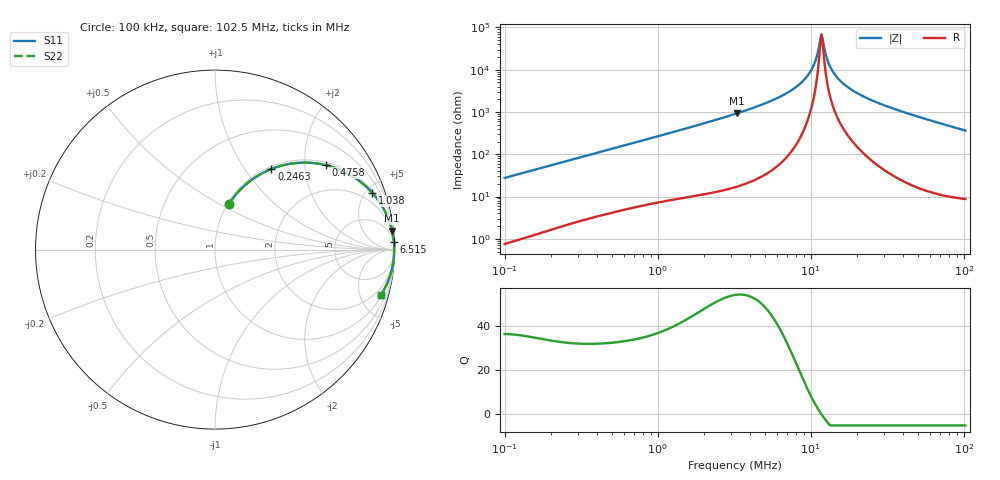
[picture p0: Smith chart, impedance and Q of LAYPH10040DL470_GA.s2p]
! LAYPH10040DL470_GA  S-PARAMETER MODEL  ( General Type )
! Model Generated by TAIYO YUDEN Corporation (http://www.ty-top.com)
! Version 1.0
! TAIYO YUDEN Control No. 180920NI43SB-FBB
! Copyright(c) 2018 TAIYO YUDEN CO.,LTD. All Rights Reserved.
! Product Description (link to TY-COMPAS)
! https://ds.yuden.co.jp/TYCOMPAS/or/detail?pn=LAYPH10040DL470MGA&u=M
! Products Name : Inductors
! Characteristics :
!  Inductance : 47 uH , SRF(min) : -Hz , DC Resistance(max) : 0.162 Ohm
!  Rated Current : Saturation :1.7 A , Temp Rise : 0.76 A (25 degC)
!  Case Size : 10.1 x 10.0 / 0.398 x 0.394 [mm/inch] , Thickness : 4 / 0.157 [mm/inch]
!  (Conditions: Temperature = 25 degC , DC Bias Current/Voltage = 0A / 0V)
! External Node Assignments :
!  1  o---GGG---o  2
! GND o---------o GND
! Frequency Range : 0.1MHz  -  102.47202MHz  [ 402 STEP ]
# MHz S RI R 50
! Freq[MHz].  S11 Real  S11 Imag  S21 Real  S21 Imag  S12 Real  S12 Imag  S22 Real  S22 Imag
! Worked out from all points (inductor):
!   401 points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, 100 kHz to 102.5 MHz, reference 50 ohm
!   read as one part in series: L = 43.7 uH near 103.5 kHz
!   highest Q = 54.3 at 3.314 MHz (marker M1), where L = 44.9 uH
!   self-resonance near 11.74 MHz
!   S11 on the Smith chart (normalised r, x): 100 kHz: 1.02, +0.55; 246.3 kHz: 1.04, +1.34; 475.8 kHz: 1.08, +2.55; 1.038 MHz: 1.15, +5.50; 6.515 MHz: 2, +49; 102.5 MHz: 1.17, -7.26
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0.1  0.0767 0.2527  0.9233 -0.2527  0.9233 -0.2527  0.0767 0.2527
0.246251  0.3147 0.4493  0.6853 -0.4493  0.6853 -0.4493  0.3147 0.4493
0.319357  0.4293 0.4796  0.5707 -0.4796  0.5707 -0.4796  0.4293 0.4796
0.475758  0.6159 0.4712  0.3841 -0.4712  0.3841 -0.4712  0.6159 0.4712
1.019889  0.8733 0.3194  0.1267 -0.3194  0.1267 -0.3194  0.8733 0.3194
1.037718  0.8769 0.3154  0.1231 -0.3154  0.1231 -0.3154  0.8769 0.3154
3.257086  0.9863 0.1074  0.0137 -0.1074  0.0137 -0.1074  0.9863 0.1074
3.314024  0.9868 0.1053  0.0132 -0.1053  0.0132 -0.1053  0.9868 0.1053
6.514629  0.9972 0.0408  0.00279 -0.0408  0.00279 -0.0408  0.9972 0.0408
8.596346  0.9984 0.0208  0.00156 -0.0208  0.00156 -0.0208  0.9984 0.0208
9.538344  0.9986 0.0137  0.00139 -0.0137  0.00139 -0.0137  0.9986 0.0137
10.22302  0.9986 0.00915  0.00136 -0.00915  0.00136 -0.00915  0.9986 0.00915
10.76858  0.9986 0.00575  0.00137 -0.00575  0.00137 -0.00575  0.9986 0.00575
11.54156  0.9986 0.00126  0.00143 -0.00126  0.00143 -0.00126  0.9986 0.00126
11.74333  0.9985 0.000148  0.00146 -0.000148  0.00146 -0.000148  0.9985 0.000148
12.1575  0.9985 -0.00208  0.00151 0.00208  0.00151 0.00208  0.9985 -0.00208
12.8063  0.9984 -0.00541  0.00161 0.00541  0.00161 0.00541  0.9984 -0.00541
13.48973  0.9983 -0.00875  0.00173 0.00875  0.00173 0.00875  0.9983 -0.00875
15.76674  0.9978 -0.0189  0.00217 0.0189  0.00217 0.0189  0.9978 -0.0189
20.80492  0.9966 -0.0381  0.00338 0.0381  0.00338 0.0381  0.9966 -0.0381
32.64791  0.9921 -0.0762  0.00794 0.0762  0.00794 0.0762  0.9921 -0.0762
102.472  0.9244 -0.2527  0.0756 0.2527  0.0756 0.2527  0.9244 -0.2527
